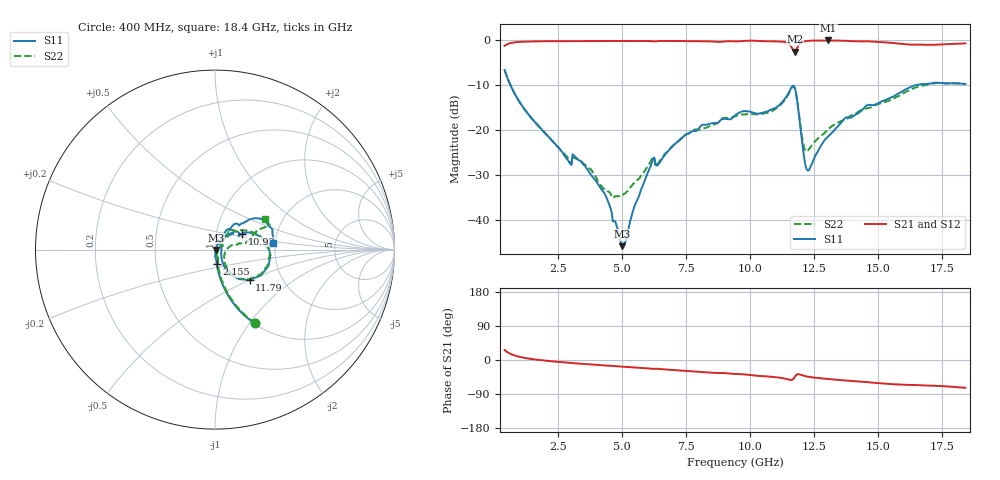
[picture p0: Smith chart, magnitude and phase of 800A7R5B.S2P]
!  American Technical Ceramics  Date:  9/12/2007
!  One Norden Lane
!  Huntington Station,  NY.  11746-2102
!  Tel:  (631) 622-4700  Fax:  (631) 622-4748
!  Part Number  800A7R5B  Mounting Orientation: Vertical
!  Description: Ultra Low ESR Microwave capacitors
!  Application: Coupling, Bypass, Tuning, DC Block
!  Filters, Matching
# GHZ S DB R 50
! Freq  |S11|  S11 Ph  |S21|  S21 Ph  |S12|  S12 Ph  |S22|  S22 Ph
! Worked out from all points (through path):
!   401 points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, 400 MHz to 18.4 GHz, reference 50 ohm
!   highest |S21| = -0.03 dB at 13.04 GHz (marker M1); lowest = -2.5 dB at 11.74 GHz (marker M2)
!   group delay of S21, straight-line fit = 12.5 ps
!   lowest |S11| = -45.8 dB at 4.99 GHz (marker M3), VSWR 1.01, Z = 50.5 - j0.176 ohm
!   |S11| at or under -10 dB: 629.9 MHz to 16.46 GHz (15.83 GHz wide, 185 % of centre)
!   |S22| runs from -35.1 to -6.6 dB; largest |S21 - S12| = 0.0017
!   S11 on the Smith chart (normalised r, x): 400 MHz: 1.01, -1.06; 2.155 GHz: 1.01, -0.17; 10.93 GHz: 1.33, +0.24; 11.79 GHz: 1.37, -0.50; 18.4 GHz: 1.95, +0.16
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0.4  -6.62 -61.8  -1.23 26.3  -1.23 26.4  -6.62 -61.4
0.94  -13.33 -76.8  -0.37 9.0  -0.37 9.0  -13.36 -75.7
2.155  -21.69 -82.6  -0.20 -2.8  -0.20 -2.8  -21.76 -78.0
2.92  -27.12 -79.8  -0.18 -7.3  -0.18 -7.3  -26.57 -69.2
3.415  -27.18 -86.5  -0.17 -10.0  -0.17 -10.0  -27.06 -72.5
4.36  -34.76 -82.7  -0.16 -14.5  -0.15 -14.5  -33.45 -50.6
4.99  -45.84 -20.0  -0.15 -17.4  -0.15 -17.4  -34.45 -6.1
6.16  -27.07 61.3  -0.18 -23.2  -0.19 -23.2  -26.34 34.5
6.43  -27.49 55.2  -0.16 -23.6  -0.16 -23.6  -27.11 41.0
7.465  -20.99 54.1  -0.17 -28.7  -0.17 -28.7  -21.17 48.5
9.4  -16.75 43.5  -0.24 -36.7  -0.25 -36.7  -16.87 49.2
10.93  -15.16 30.6  -0.23 -45.0  -0.23 -45.0  -15.46 39.4
11.47  -11.95 18.2  -0.67 -51.2  -0.67 -51.2  -12.17 21.0
11.74  -10.66 -29.5  -2.50 -44.0  -2.50 -44.0  -10.74 -28.1
11.785  -11.82 -41.4  -2.18 -39.7  -2.19 -39.8  -11.88 -39.9
12.145  -27.68 -33.8  -0.21 -42.5  -0.21 -42.5  -24.47 -28.0
12.415  -27.27 29.7  -0.07 -45.7  -0.07 -45.7  -23.27 4.7
13.045  -21.40 56.2  -0.03 -50.2  -0.04 -50.2  -19.82 15.8
13.72  -17.22 56.3  -0.10 -54.3  -0.11 -54.2  -17.67 12.7
15.43  -12.90 42.6  -0.52 -63.2  -0.52 -63.2  -13.41 19.0
16.555  -9.88 29.4  -0.95 -66.4  -0.95 -66.5  -10.34 24.2
18.4  -9.74 6.6  -0.69 -73.3  -0.69 -73.3  -9.68 31.2
